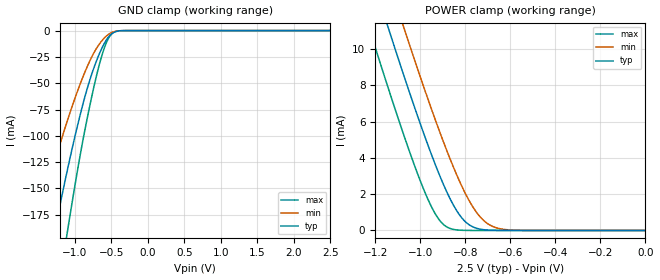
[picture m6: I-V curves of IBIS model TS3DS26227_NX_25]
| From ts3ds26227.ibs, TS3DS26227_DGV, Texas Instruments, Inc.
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[Model]   TS3DS26227_NX_25
Model_type  Terminator
| variable   typ   min   max
C_comp   2.63pF   2.34pF   2.97pF
| C_tri-state   2.63pF   2.34pF   2.97pF
[Temperature Range]   40   100   -40
| Ambient temperature   25   85   -40
[Voltage range]   2.5   2.3   2.7
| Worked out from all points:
|   GND clamp passes 1 mA (typ) near -0.44 V on its own axis
|   POWER clamp passes 1 mA (typ) near -0.83 V on its own axis
[GND Clamp]
| TS3DS26227_NX_25
|   Voltage   I(typ)   I(min)   I(max)
-2.5V     -683.9mA   -490.2mA   -863.9mA
-1.55V    -291.6mA   -195.5mA   -398.4mA
-1.515V   -278.3mA   -186.1mA   -381.7mA
-1.28V    -192.5mA   -126.2mA   -271.6mA
-1.25V    -182.1mA   -119.1mA   -257.9mA
-1.095V   -130.5mA   -84.26mA   -188.6mA
-920mV    -78.41mA   -49.69mA   -116.1mA
-755mV    -38.79mA   -23.36mA   -58.77mA
-620mV    -15.49mA   -8.937mA   -21.76mA
-515mV    -4.325mA   -2.602mA   -4.823mA
-355mV    -126.4uA   -109.9uA   -61.18uA
2.5V      3.489nA    8.419nA    200.2pA
[POWER Clamp]
| TS3DS26227_NX_25
|   Voltage   I(typ)   I(min)   I(max)
-2.5V     67.33mA    69.82mA    64.3mA
-1.245V   15.22mA    17.89mA    11.89mA
-1.21V    13.84mA    16.5mA     10.5mA
-1.15V    11.49mA    14.15mA    8.16mA
-1.125V   10.53mA    13.19mA    7.204mA
-1.075V   8.634mA    11.28mA    5.339mA
-975mV    5.025mA    7.58mA     1.983mA
-910mV    2.924mA    5.324mA    501.7uA
-810mV    618.6uA    2.304mA    9.382uA
-710mV    34.34uA    462.1uA    106.4nA
-600mV    893.6nA    27.97uA    1.131nA
-31.15fV  3.489nA    7.774nA    234.2pA
